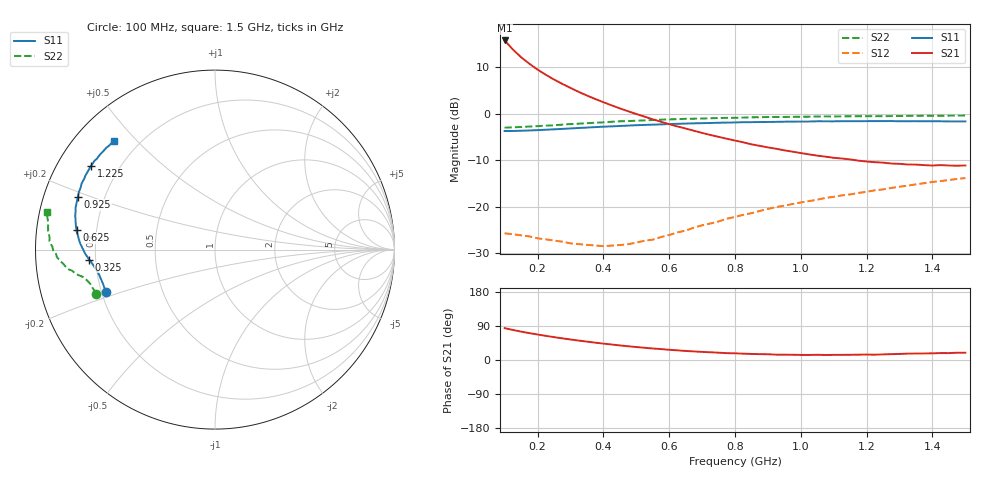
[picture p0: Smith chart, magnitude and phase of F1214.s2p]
! Date: Tue Apr 09 10:03:22 1996
# MHZ  S  MA  R  50.0000
!  POLYFET RF DEVICES
!  F1214
!  S PARAMETERS
!  VDS=12.5V, IDQ=400mA
!FREQ  S11MAG S11ANG S21MAG S21ANG S12MAG S12ANG S22MAG S22ANG
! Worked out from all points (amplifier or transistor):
!   57 points, 100 MHz to 1.5 GHz, reference 50 ohm
!   highest |S21| = 15.8 dB at 100 MHz (marker M1)
!   |S21| within 3 dB of that: start of sweep to 140.8 MHz
!   unconditionally stable (mu >= 1): 287 MHz to 743.6 MHz
!   at 325 MHz: K = 1.15, MAG = 14.0 dB, |S12| = -28.1 dB
!   at 800 MHz: K = 0.94, MSG = 8.2 dB, |S12| = -22.2 dB
!   at 1.5 GHz: K = 0.79, MSG = 1.4 dB, |S12| = -13.9 dB
!   S11 on the Smith chart (normalised r, x): 100 MHz: 0.22, -0.18; 325 MHz: 0.17, -0.04; 625 MHz: 0.12, +0.07; 925 MHz: 0.10, +0.18; 1.225 GHz: 0.10, +0.30; 1.5 GHz: 0.11, +0.43
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100  0.6523 -158.8  6.164 84.2  0.05149 7.2  0.7078 -159.8
125  0.6524 -163.0  4.929 79.3  0.0504 5.7  0.7145 -162.7
150  0.6564 -165.7  4.067 74.9  0.04896 5.4  0.7204 -164.6
175  0.6604 -167.8  3.463 70.9  0.04773 5.1  0.728 -165.8
200  0.6662 -169.4  2.995 67.3  0.04552 5.5  0.736 -166.8
225  0.6731 -170.8  2.632 63.8  0.04437 6.8  0.7434 -167.7
250  0.6797 -172.0  2.34 60.3  0.04305 7.9  0.7525 -168.3
275  0.6866 -173.2  2.1 57.2  0.04185 10.2  0.7639 -168.9
325  0.7026 -175.5  1.721 51.2  0.03937 15.8  0.7817 -170.0
350  0.7099 -176.4  1.573 48.5  0.03868 18.1  0.7922 -170.5
400  0.726 -178.6  1.333 43.2  0.03744 27.1  0.8084 -171.8
450  0.7385 179.4  1.143 38.5  0.03848 34.7  0.8297 -172.8
500  0.7526 177.3  0.994 34.3  0.04087 44.1  0.8415 -173.9
575  0.7679 174.1  0.8209 28.8  0.04694 53.8  0.864 -175.7
625  0.7794 171.9  0.7305 25.4  0.05268 58.7  0.8747 -176.7
700  0.7923 168.7  0.6219 21.4  0.06283 63.4  0.8881 -178.8
800  0.8058 164.5  0.5144 17.6  0.07736 65.7  0.905 179.2
925  0.8183 159.0  0.4199 14.2  0.09882 66.7  0.9238 176.6
1050  0.8296 153.6  0.3539 13.7  0.1187 64.6  0.9346 174.1
1225  0.8333 145.8  0.3007 14.1  0.1498 61.3  0.9429 171.1
1275  0.8342 143.6  0.2909 15.5  0.1587 60.7  0.9439 170.3
1500  0.8262 133.2  0.2772 19.2  0.2028 53.4  0.958 167.3
